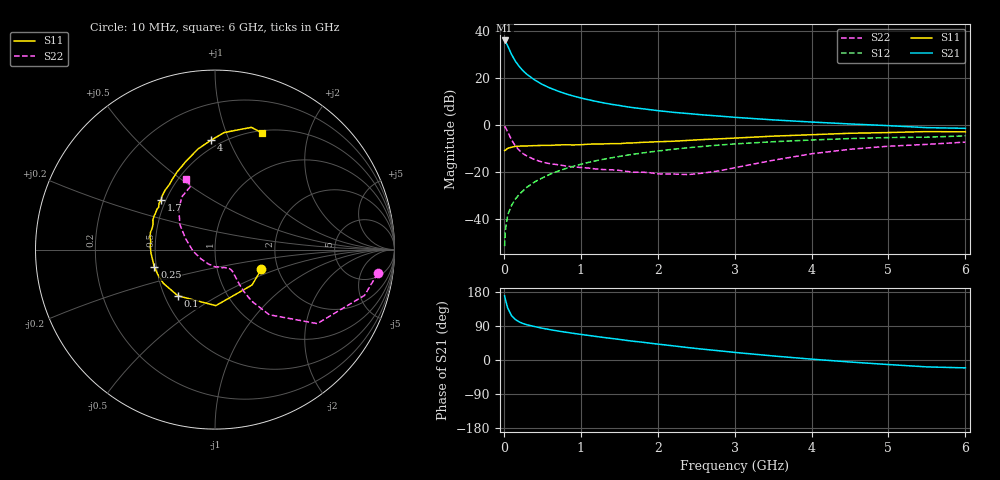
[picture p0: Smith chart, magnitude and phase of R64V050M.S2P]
! SIEMENS Small Signal Semiconductors
! BFR193
! Si NPN RF Bipolar Junction Transistor in SOT23
! VCE = 4 V  IC = 50 mA
! Common Emitter S-Parameters:  May  1996
# GHz  S  MA  R  50
!  f  S11  S21  S12  S22
! GHz  MAG  ANG  MAG  ANG  MAG  ANG  MAG  ANG
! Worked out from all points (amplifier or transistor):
!   36 points, 10 MHz to 6 GHz, reference 50 ohm
!   highest |S21| = 35.8 dB at 10 MHz (marker M1)
!   |S21| within 3 dB of that: start of sweep to 59.64 MHz
!   unconditionally stable (mu >= 1): 404.5 MHz to 1.867 GHz
!   at 250 MHz: K = 0.95, MSG = 25.5 dB, |S12| = -28.1 dB
!   at 1.4 GHz: K = 1.02, MAG = 10.5 dB, |S12| = -14.1 dB
!   at 6 GHz: K = 0.95, MSG = 1.6 dB, |S12| = -4.8 dB
!   S11 on the Smith chart (normalised r, x): 10 MHz: 1.64, -0.39; 100 MHz: 0.59, -0.34; 250 MHz: 0.49, -0.11; 1.7 GHz: 0.47, +0.32; 4 GHz: 0.44, +0.86; 6 GHz: 0.53, +1.35
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0.01  0.2809 -22.8  61.5 169.5  0.0026 83.2  0.9161 -8.3
0.02  0.2854 -43.7  58.8 159.7  0.0056 84.3  0.8715 -17.0
0.05  0.3123 -89.2  47.19 137.3  0.012 68.9  0.7032 -35.9
0.1  0.3301 -128.8  31.09 117.1  0.0191 68.6  0.4726 -50.2
0.15  0.3437 -146.9  22.26 106.6  0.0261 70.5  0.3515 -54.6
0.2  0.348 -156.8  17.24 100.5  0.0328 72.0  0.284 -55.4
0.25  0.3516 -164.0  13.92 96.2  0.0393 72.9  0.2405 -55.0
0.3  0.3518 -169.1  11.72 93.0  0.0466 74.0  0.2144 -54.2
0.4  0.3571 -176.9  8.911 88.2  0.0604 74.6  0.1802 -52.7
0.5  0.3608 177.3  7.148 83.9  0.0735 74.3  0.1592 -51.4
0.6  0.3606 173.1  5.999 80.1  0.088 73.6  0.1475 -51.3
0.7  0.3686 169.1  5.184 76.6  0.1017 72.7  0.1404 -51.7
0.8  0.3723 164.9  4.541 73.5  0.1158 71.4  0.1323 -52.9
1.1  0.3827 154.8  3.372 64.9  0.1571 67.9  0.1189 -58.8
1.4  0.3941 145.2  2.697 56.9  0.1968 63.7  0.1095 -67.6
1.7  0.4091 137.0  2.272 49.1  0.2359 59.4  0.0969 -80.5
2.2  0.4423 125.2  1.827 37.4  0.2988 51.7  0.0888 -112.3
3.5  0.568 99.7  1.26 10.7  0.432 31.2  0.1744 159.7
4  0.6091 92.2  1.133 2.3  0.4703 24.2  0.2397 144.6
4.5  0.6537 85.6  1.032 -5.3  0.5048 17.1  0.2986 132.4
5.5  0.7107 73.4  0.861 -18.2  0.5406 3.4  0.3798 110.6
6  0.7009 67.9  0.833 -20.8  0.5751 -0.6  0.4239 112.8
